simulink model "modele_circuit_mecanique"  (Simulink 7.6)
settings: Solver=ode45  StartTime=0.0  StopTime=1  RelTol=1e-3
InitFcn:
  | clc
  | k2=2000;
  | f2=500;
  | m2=10;
  | 
  | m1=5;
  | k1=5000;
  | f1=1000;
StopFcn:
  | close all
  | load pos_vit.mat
  | plotyy(pv(1,:),pv(2,:),pv(1,:),pv(3,:))
  | title('Vitesse et position de la masse 2')
  | xlabel('temps')
  | grid

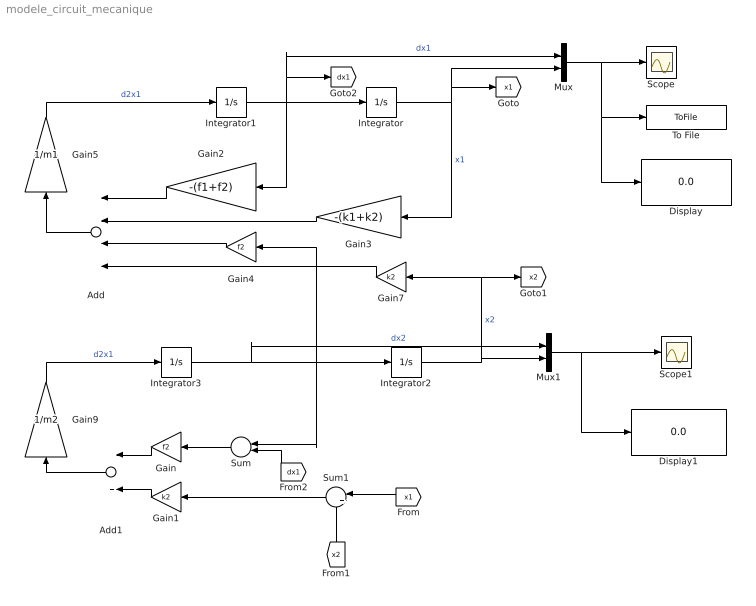
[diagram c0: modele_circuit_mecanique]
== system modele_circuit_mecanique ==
  Add : Sum  Inputs=4
  Add1 : Sum  Inputs=2
  Display : Display
  Display1 : Display
  Gain : Gain  Gain=f2
  Gain1 : Gain  Gain=k2
  Gain2 : Gain  Gain=-(f1+f2)
  Gain3 : Gain  Gain=-(k1+k2)
  Gain4 : Gain  Gain=f2
  Gain5 : Gain  Gain=1/m1
  Gain7 : Gain  Gain=k2
  Gain9 : Gain  Gain=1/m2
  Integrator : Integrator
  Integrator1 : Integrator  InitialCondition=1
  Integrator2 : Integrator
  Integrator3 : Integrator  InitialCondition=10
  Mux : Mux  Inputs=2
  Mux1 : Mux  Inputs=2
  Scope : Scope
  Scope1 : Scope
  Sum : Sum  Inputs=|-+
  Sum1 : Sum  Inputs=|+-
  To File : ToFile  Filename=pos_vit.mat  MatrixName=pv
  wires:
  Integrator1/1 -> Integrator/1, Gain2/1, [dx1], Mux/1  "dx1"
  Integrator3/1 -> Integrator2/1, Gain4/1, Sum/1, Mux1/1  "dx2"
  Integrator/1 -> Gain3/1, [x1], Mux/2  "x1"
  Integrator2/1 -> Gain7/1, [x2], Mux1/2  "x2"
  Gain2/1 -> Add/1
  Gain3/1 -> Add/2
  Gain4/1 -> Add/3
  Gain7/1 -> Add/4
  Add/1 -> Gain5/1
  Gain5/1 -> Integrator1/1  "d2x1"
  Gain9/1 -> Integrator3/1  "d2x1"
  Gain/1 -> Add1/1
  Sum/1 -> Gain/1
  Gain1/1 -> Add1/2
  Sum1/1 -> Gain1/1
  Add1/1 -> Gain9/1
  [x1] -> Sum1/1
  [x2] -> Sum1/2
  [dx1] -> Sum/2
  Mux/1 -> Scope/1, To File/1, Display/1
  Mux1/1 -> Scope1/1, Display1/1
